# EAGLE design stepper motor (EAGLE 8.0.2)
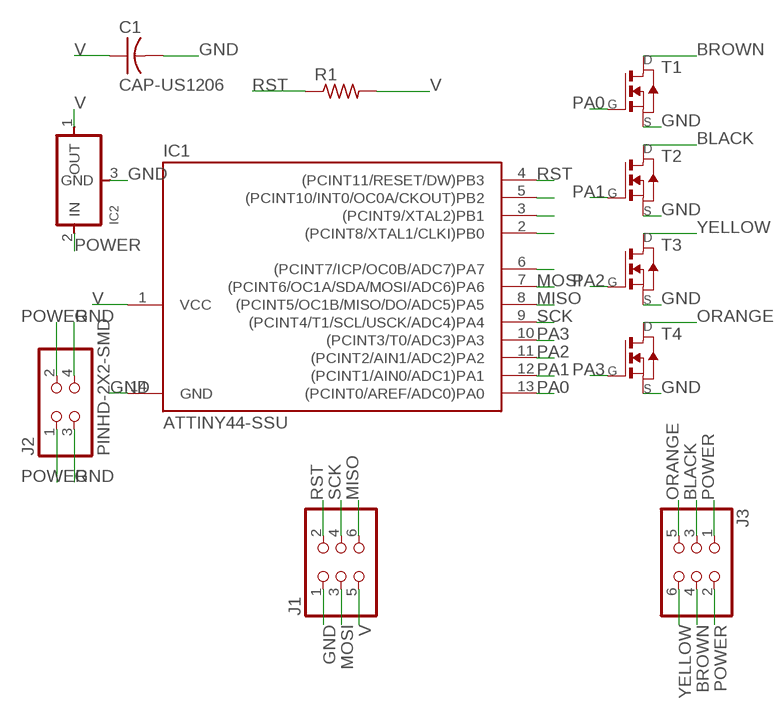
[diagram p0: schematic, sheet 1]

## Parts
C1  CAP-US1206  [C1206]
IC1  ATTINY44-SSU  [SOIC14]
IC2  REGULATORSOT23  [SOT23]
J1  PINHD-2X3-SMD  [2X03SMD]
J2  PINHD-2X2-SMD  [2X02SMD]
J3  PINHD-2X3-SMD  [2X03SMD]
R1  RES-US1206  [R1206]
T1  NMOSFETSOT23  [SOT-23]
T2  NMOSFETSOT23  [SOT-23]
T3  NMOSFETSOT23  [SOT-23]
T4  NMOSFETSOT23  [SOT-23]

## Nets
BLACK: J3.3 T2.1(D)
BROWN: J3.4 T1.1(D)
GND: C1.2 IC1.14(GND) IC2.3(GND) J1.1 J2.3 J2.4 T1.2(S) T2.2(S) T3.2(S) T4.2(S)
MISO: IC1.8((PCINT5/OC1B/MISO/DO/ADC5)PA5) J1.6
MOSI: IC1.7((PCINT6/OC1A/SDA/MOSI/ADC6)PA6) J1.3
N$2: IC1.5((PCINT10/INT0/OC0A/CKOUT)PB2)
N$3: IC1.3((PCINT9/XTAL2)PB1)
N$4: IC1.2((PCINT8/XTAL1/CLKI)PB0)
N$5: IC1.6((PCINT7/ICP/OC0B/ADC7)PA7)
ORANGE: J3.5 T4.1(D)
PA0: IC1.13((PCINT0/AREF/ADC0)PA0) T1.3(G)
PA1: IC1.12((PCINT1/AIN0/ADC1)PA1) T2.3(G)
PA2: IC1.11((PCINT2/AIN1/ADC2)PA2) T3.3(G)
PA3: IC1.10((PCINT3/T0/ADC3)PA3) T4.3(G)
POWER: IC2.2(IN) J2.1 J2.2 J3.1 J3.2
RST: IC1.4((PCINT11/RESET/DW)PB3) J1.2 R1.1
SCK: IC1.9((PCINT4/T1/SCL/USCK/ADC4)PA4) J1.4
V: C1.1 IC1.1(VCC) IC2.1(OUT) J1.5 R1.2
YELLOW: J3.6 T3.1(D)

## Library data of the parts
C1 = fab:CAP-US
IC1 = fab:ATTINY44
IC2 = fab:REGULATOR
J1 J3 = fab:PINHD-2X3-SMD: PIN HEADER
J2 = fab:PINHD-2X2-SMD
R1 = fab:RES-US: Resistor (US Symbol)
T1-T4 = fab:NMOSFET: MOS FET

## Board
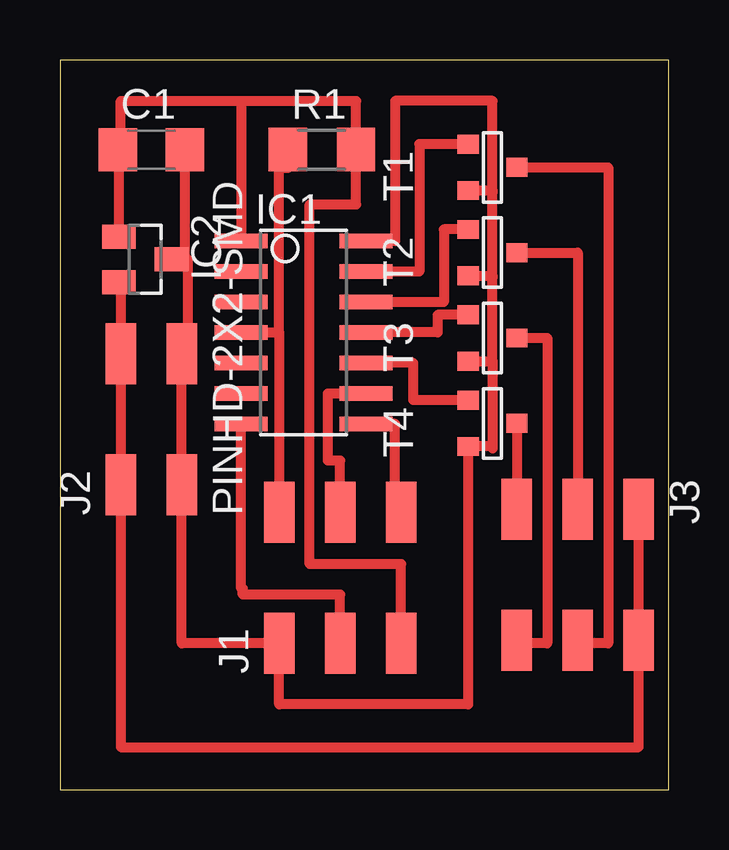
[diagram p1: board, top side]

Size 25.38 x 30.4 mm. Coordinates in mm from the lower left corner, seen from the top.
Outline: 0,0 25.38,0 25.38,30.4 0,30.4 0,0
Copper layers (1*16): Top 0.035mm / dielectric 1.5mm / Bottom 0.035mm
Design rules "default": minimum track width 10mil, minimum drill 24mil, track to track 8mil, track to pad 8mil, pad to pad 8mil, via to via 8mil, smd to smd 8mil, copper to edge 40mil, drill to drill 8mil, minimum pad ring 10mil, minimum via ring 8mil, stop-mask expansion 4mil, vias tented up to drill 0mil, thermal gap 10mil

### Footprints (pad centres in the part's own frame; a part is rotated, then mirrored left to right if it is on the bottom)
C1206 = smd 1.6 x 1.8: 1 -1.4,0; 2 1.4,0
SOIC14 = smd 0.61 x 2.21: 1 -3.81,-2.603; 2 -2.54,-2.603; 3 -1.27,-2.603; 4 0,-2.603; 5 1.27,-2.603; 6 2.54,-2.603; 7 3.81,-2.603; 8 3.81,2.603; 9 2.54,2.603; 10 1.27,2.603; 11 0,2.603; 12 -1.27,2.603; 13 -2.54,2.603; 14 -3.81,2.603
SOT23 = smd 1 x 1.4: 1 -0.95,-1.1; 2 0.95,-1.1; 3 0,1.1
2X03SMD = smd 2.54 x 1.27: 1 -2.54,2.54; 2 2.92,2.54; 3 -2.54,0; 4 2.92,0; 5 -2.54,-2.54; 6 2.92,-2.54
2X02SMD = smd 2.54 x 1.27: 1 -2.54,1.27; 2 2.92,1.27; 3 -2.54,-1.27; 4 2.92,-1.27
R1206 = smd 1.6 x 1.803: 1 -1.422,0; 2 1.422,0
SOT-23 = smd 0.787 x 0.889: 1 0.025,-1.016; 2 -0.94,1.016; 3 0.991,1.016

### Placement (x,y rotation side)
C1  3.81,26.67 0 top
IC1  10.16,19.05 270 top
IC2  3.56,22.1 270 top
J1  11.68,8.64 90 top
J2  3.81,15.24 90 top
J3  21.59,9.14 270 top
R1  10.92,26.67 0 top
T1  18.03,25.91 90 top
T2  18.03,22.35 90 top
T3  18.03,18.8 90 top
T4  18.03,15.24 90 top

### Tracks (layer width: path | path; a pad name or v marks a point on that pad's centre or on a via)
BLACK
  Top 0.406: T2.1 21.59,22.38 J3.3
BROWN
  Top 0.406: T1.1 22.86,25.93 22.86,6.1 21.59,6.1 J3.4
GND
  Top 0.406: 18.03,14.3 T4.2 17.02,3.56 9.14,3.56 J1.1 5.08,6.1 J2.3 J2.4 5.33,18.16 5.33,22.1 IC2.3 5.21,22.1 C1.2 | 18.03,14.3 18.03,14.22 | 18.03,21.34 18.03,24.89 | 18.03,17.78 18.03,21.34 | 18.03,17.78 18.03,14.3 | 18.03,24.89 18.03,28.7 13.97,28.7 13.97,22.86 IC1.14 | T1.2 18.03,24.97 18.03,24.89 | T2.2 18.03,21.41 18.03,21.34 | T3.2 18.03,17.86 18.03,17.78
MISO
  Top 0.406: J1.6 13.97,11.56 13.97,15.24 IC1.8
MOSI
  Top 0.406: J1.3 11.68,8.13 7.62,8.13 7.62,8.38 7.56,8.38 IC1.7
ORANGE
  Top 0.406: T4.1 J3.5
PA0
  Top 0.406: T1.3 14.99,26.9 14.99,21.59 IC1.13
PA1
  Top 0.406: T2.3 16,23.34 16,20.32 IC1.12
PA2
  Top 0.406: T3.3 15.75,19.79 15.75,19.05 IC1.11
PA3
  Top 0.406: T4.3 14.73,16.23 14.73,17.78 IC1.10
POWER
  Top 0.406: 2.46,12.7 J2.1 | 2.46,18.16 J2.2 | IC2.2 2.54,21.15 J2.2 | J2.2 J2.1 | J2.1 2.54,1.78 24.13,1.78 J3.2 J3.1
RST
  Top 0.406: IC1.4 9.14,19.05 | 9.14,19.05 9.14,25.91 9.5,25.91 R1.1 | 9.14,19.05 J1.2
SCK
  Top 0.406: J1.4 11.68,13.72 11.18,13.72 11.18,16.51 IC1.9
V
  Top 0.406: IC2.1 2.46,26.67 C1.1 2.54,26.67 2.54,28.7 7.56,28.7 | 7.56,28.7 12.34,28.7 R1.2 12.34,24.38 10.41,24.38 10.41,9.4 14.22,9.4 J1.5 | 7.56,28.7 IC1.1
YELLOW
  Top 0.406: T3.1 20.32,18.82 20.32,6.1 19.05,6.1 J3.6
